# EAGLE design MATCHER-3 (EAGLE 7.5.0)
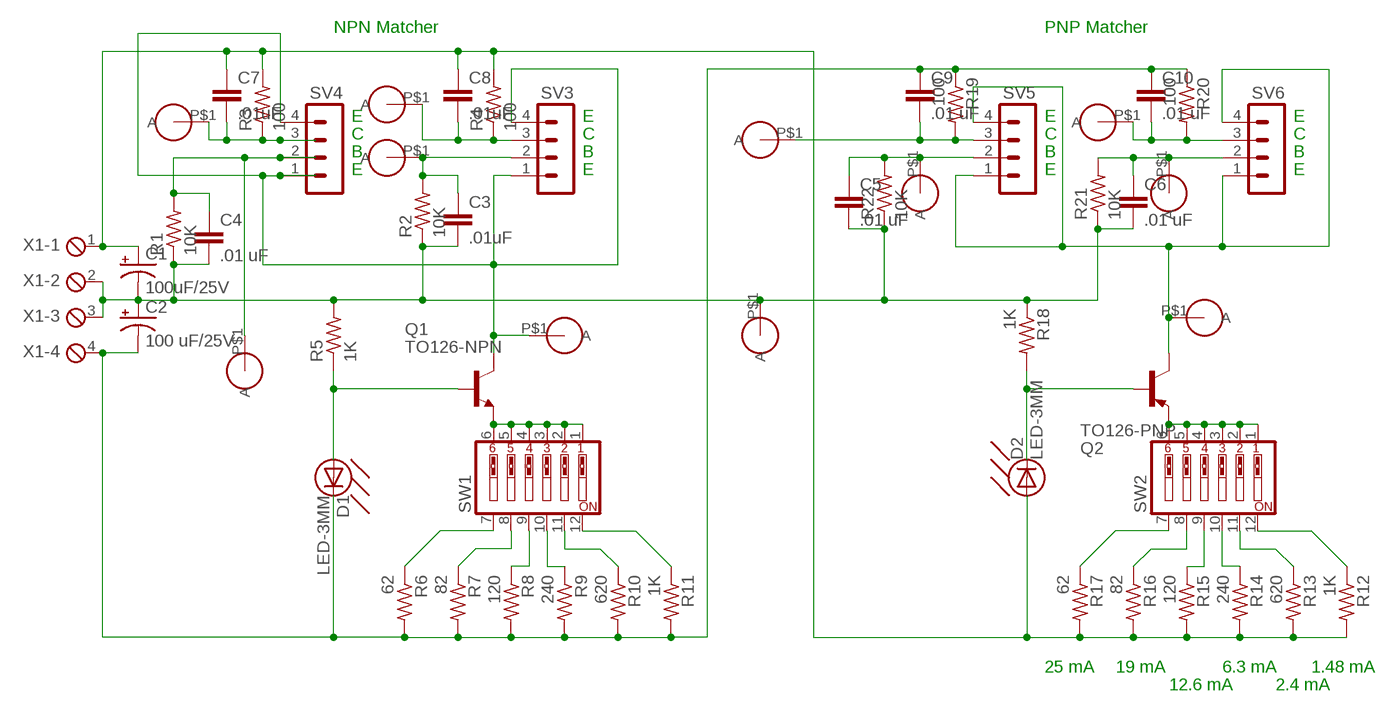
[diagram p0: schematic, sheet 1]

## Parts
C1  100uF/25V  CAP-POL-5/10  [CAP-POL-5/10]
C2  100 uF/25V  CAP-POL-5/10  [CAP-POL-5/10]
C3  .01uF  C5/2.5  [C5B2.5]
C4  .01 uF  C5/2.5  [C5B2.5]
C5  .01 uF  C5/2.5  [C5B2.5]
C6  .01 uF  C5/2.5  [C5B2.5]
C7  .01uF  C5/2.5  [C5B2.5]
C8  .01uF  C5/2.5  [C5B2.5]
C9  .01 uF  C5/2.5  [C5B2.5]
C10  .01 uF  C5/2.5  [C5B2.5]
D1  LED-3MM  [LED3MM]
D2  LED-3MM  [LED3MM]
GND  TESTPOINT  [TEST]
Q1  TO126-NPN  [TO126]
Q2  TO126-PNP  [TO126]
R1  10K  RESISTOR-1/4W  [FILM-RESISTOR]
R2  10K  RESISTOR-1/4W  [FILM-RESISTOR]
R3  100  RESISTOR-1/4W  [FILM-RESISTOR]
R4  100  RESISTOR-1/4W  [FILM-RESISTOR]
R5  1K  RESISTOR-1/4W  [FILM-RESISTOR]
R6  62  RESISTOR-1/4W  [FILM-RESISTOR]
R7  82  RESISTOR-1/4W  [FILM-RESISTOR]
R8  120  RESISTOR-1/4W  [FILM-RESISTOR]
R9  240  RESISTOR-1/4W  [FILM-RESISTOR]
R10  620  RESISTOR-1/4W  [FILM-RESISTOR]
R11  1K  RESISTOR-1/4W  [FILM-RESISTOR]
R12  1K  RESISTOR-1/4W  [FILM-RESISTOR]
R13  620  RESISTOR-1/4W  [FILM-RESISTOR]
R14  240  RESISTOR-1/4W  [FILM-RESISTOR]
R15  120  RESISTOR-1/4W  [FILM-RESISTOR]
R16  82  RESISTOR-1/4W  [FILM-RESISTOR]
R17  62  RESISTOR-1/4W  [FILM-RESISTOR]
R18  1K  RESISTOR-1/4W  [FILM-RESISTOR]
R19  100  RESISTOR-1/4W  [FILM-RESISTOR]
R20  100  RESISTOR-1/4W  [FILM-RESISTOR]
R21  10K  RESISTOR-1/4W  [FILM-RESISTOR]
R22  10K  RESISTOR-1/4W  [FILM-RESISTOR]
SV3  MA04-1  [MA04-1]
SV4  MA04-1  [MA04-1]
SV5  MA04-1  [MA04-1]
SV6  MA04-1  [MA04-1]
SW1  SW_DIP-6  [EDG-06]
SW2  SW_DIP-6  [EDG-06]
VB-A-N  TESTPOINT  [TEST]
VB-A-P  TESTPOINT  [TEST]
VB-B-N  TESTPOINT  [TEST]
VB-B-P  TESTPOINT  [TEST]
VC-A-N  TESTPOINT  [TEST]
VC-A-P  TESTPOINT  [TEST]
VC-B-N  TESTPOINT  [TEST]
VC-B-P  TESTPOINT  [TEST]
VE-N  TESTPOINT  [TEST]
VE-P  TESTPOINT  [TEST]
X1  MPT4  [4POL254]

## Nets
GND: C1.P$2(-) C2.P$1(+) C3.2 C4.2 C5.2 C6.2 GND.P$1(A) R1.P$1 R2.P$1 R5.P$2 R18.P$1 R21.P$1 R22.P$1 X1.2 X1.3
N$1: Q1.1(E) SW1.1 SW1.2 SW1.3 SW1.4 SW1.5 SW1.6
N$2: R6.P$1 SW1.7
N$3: R11.P$1 SW1.12
N$4: R8.P$1 SW1.9
N$5: R7.P$1 SW1.8
N$6: R9.P$1 SW1.10
N$7: R10.P$1 SW1.11
N$8: C5.1 R22.P$2 SV5.2 VB-A-P.P$1(A)
N$9: R15.P$1 SW2.9
N$10: D1.P$1-A(A) Q1.3(B) R5.P$1
N$11: Q1.2(C) SV3.1 SV3.4 SV4.1 SV4.4 VE-N.P$1(A)
N$12: C9.2 R19.P$2 SV5.3 VC-A-P.P$1(A)
N$13: C3.1 R2.P$2 SV3.2 VB-B-N.P$1(A)
N$14: C7.2 R3.P$1 SV4.3 VC-A-N.P$1(A)
N$15: C4.1 R1.P$2 SV4.2 VB-A-N.P$1(A)
N$16: C8.2 R4.P$1 SV3.3 VC-B-N.P$1(A)
N$17: C1.P$1(+) C7.1 C8.1 D2.P$1-A(A) R3.P$2 R4.P$2 R12.P$2 R13.P$2 R14.P$2 R15.P$2 R16.P$2 R17.P$2 X1.1
N$18: R14.P$1 SW2.10
N$19: R13.P$1 SW2.11
N$20: R12.P$1 SW2.12
N$21: R17.P$1 SW2.7
N$22: R16.P$1 SW2.8
N$23: Q2.1(E) SW2.1 SW2.2 SW2.3 SW2.4 SW2.5 SW2.6
N$26: C2.P$2(-) C9.1 C10.1 D1.P$2-C(C) R6.P$2 R7.P$2 R8.P$2 R9.P$2 R10.P$2 R11.P$2 R19.P$1 R20.P$1 X1.4
N$27: C6.1 R21.P$2 SV6.2 VB-B-P.P$1(A)
N$28: C10.2 R20.P$2 SV6.3 VC-B-P.P$1(A)
N$29: Q2.2(C) SV5.1 SV5.4 SV6.1 SV6.4 VE-P.P$1(A)
N$32: D2.P$2-C(C) Q2.3(B) R18.P$2

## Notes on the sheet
- NPN Matcher | PNP Matcher
- E | E | E | E
- C | C | C | C
- B | B | B | B
- E | E | E | E
- 25 mA | 19 mA | 6.3 mA | 1.48 mA
- 12.6 mA | 2.4 mA

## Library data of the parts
C1 C2 = ADC Project:CAP-POL-5/10
C3-C10 = capacitor-wima:C: CAPACITOR
D1 D2 = Adcom Project:LED-3MM
GND VB-A-N VB-A-P VB-B-N VB-B-P VC-A-N VC-A-P VC-B-N VC-B-P VE-N VE-P = Adcom Project:TESTPOINT
Q1 = Adcom Project:TO126-NPN
Q2 = Adcom Project:TO126-PNP
R1-R22 = ADC Project:RESISTOR-1/4W: 1/4 Watt Resistor
SV3-SV6 = con-lstb:MA04-1: PIN HEADER; OC_FARNELL: unknown; OC_NEWARK: unknown
SW1 SW2 = special:SW_DIP-6: DIP SWITCH
X1 = con-phoenix-254:MPT4: PHOENIX CONNECTOR; OC_FARNELL: unknown; OC_NEWARK: unknown

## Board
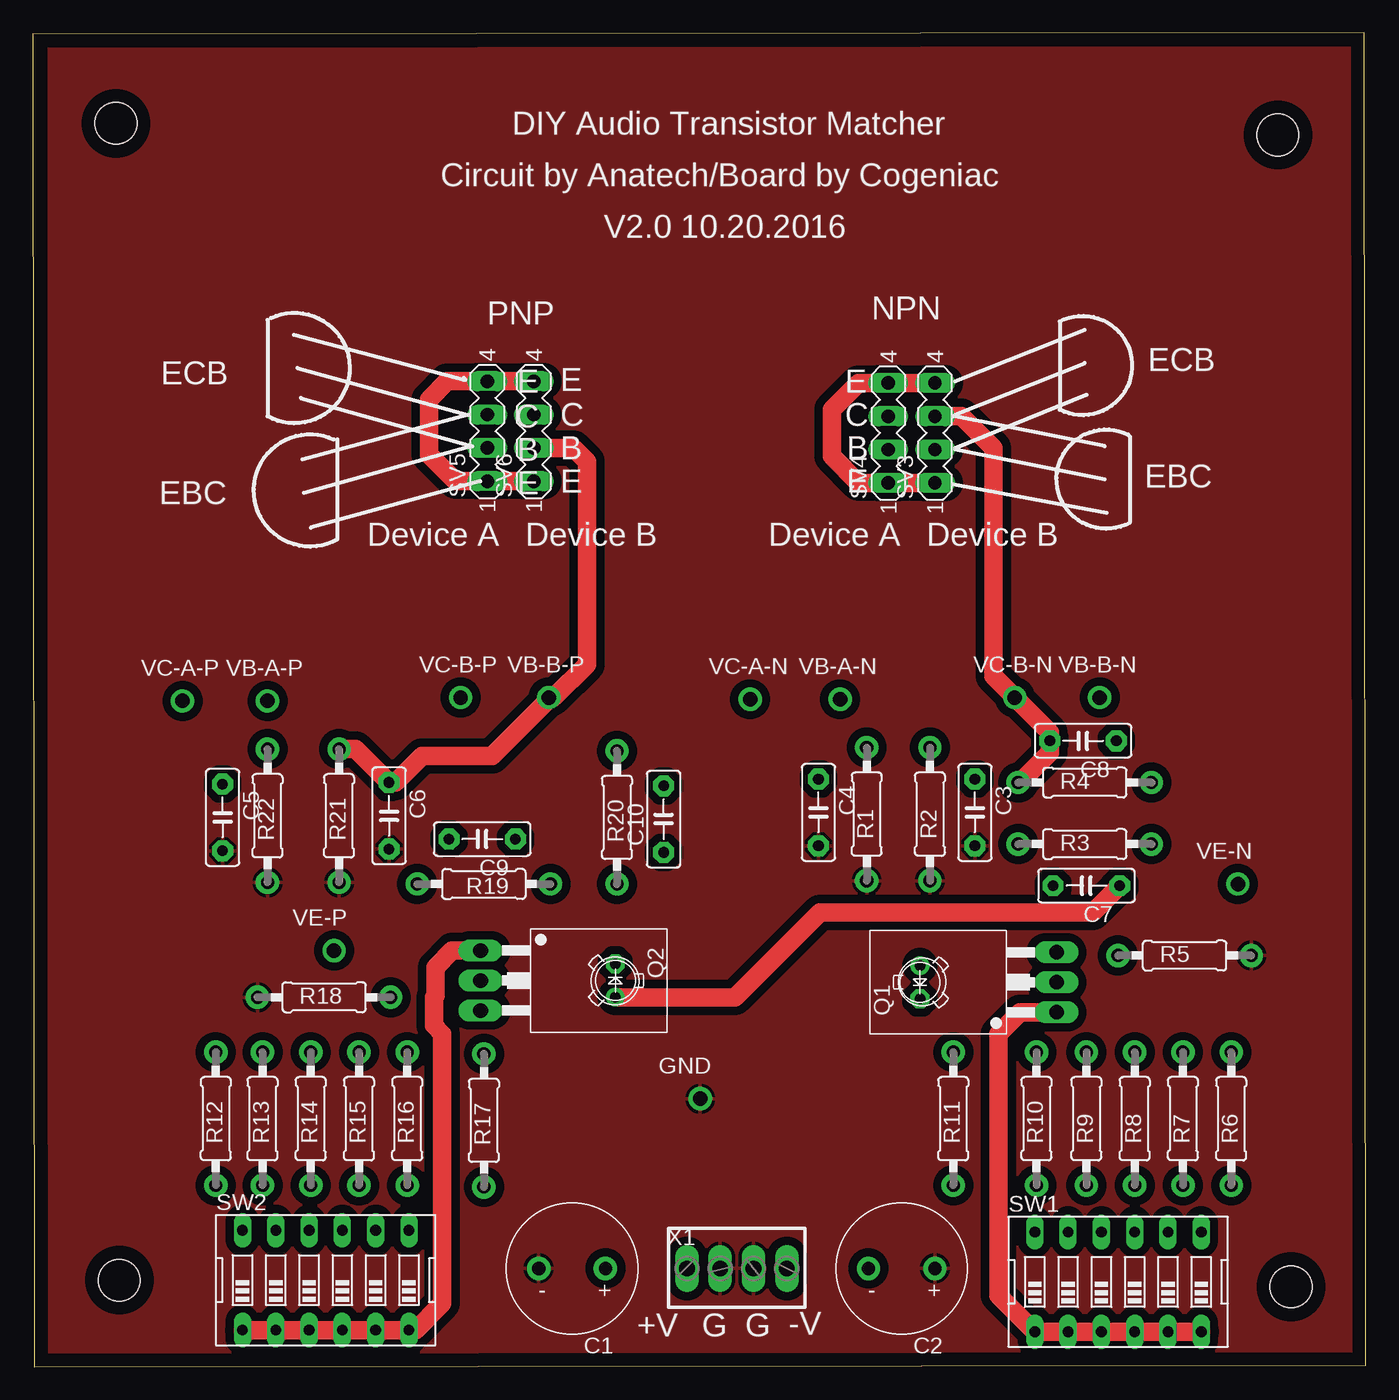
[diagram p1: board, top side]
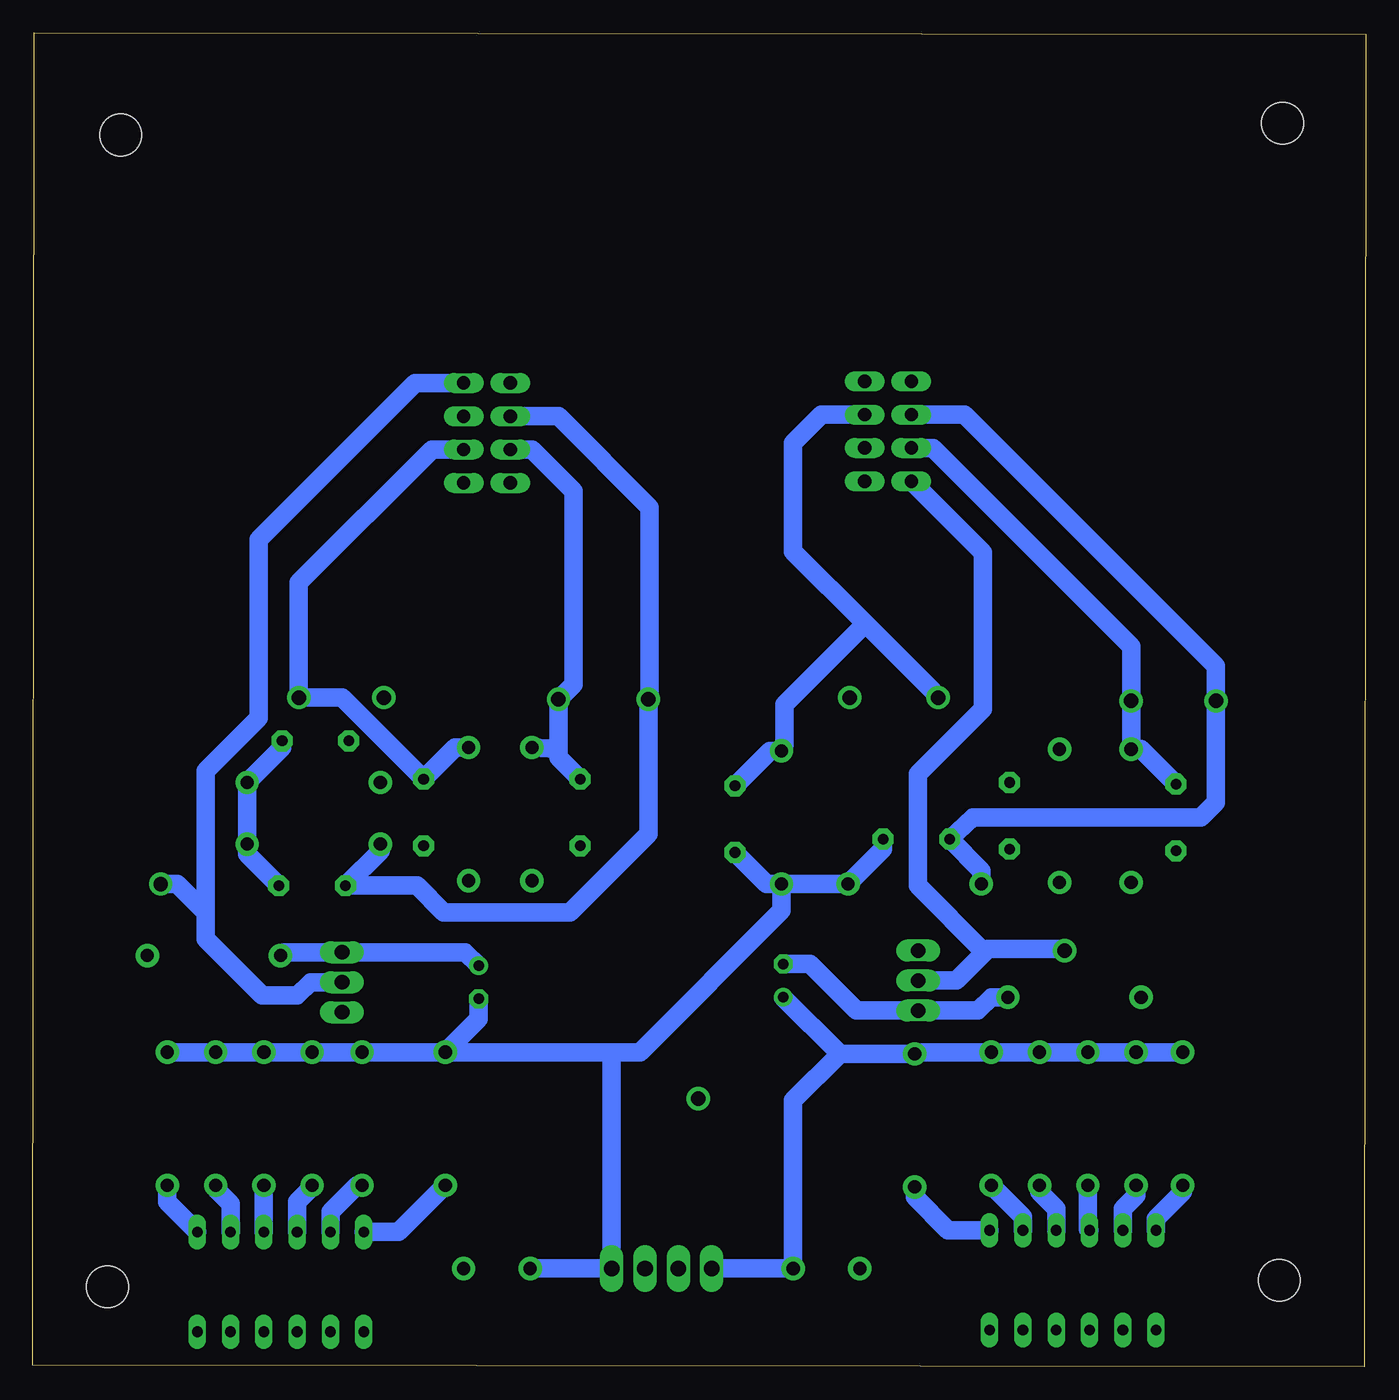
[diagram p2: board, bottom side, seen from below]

Size 101.71 x 101.78 mm. Coordinates in mm from the lower left corner, seen from the top.
Outline: 0.13,0 101.71,0.13 101.58,101.78 0,101.65 0.13,0
Copper layers (1*16): Top 0.035mm / dielectric 1.5mm / Bottom 0.035mm
Design rules "default *": minimum track width 56mil, minimum drill 24mil, track to track 25mil, track to pad 15mil, pad to pad 15mil, via to via 8mil, smd to smd 8mil, copper to edge 40mil, drill to drill 8mil, minimum pad ring 10mil, minimum via ring 8mil, stop-mask expansion 4mil, vias tented up to drill 0mil, thermal gap 10mil
Holes 3.2 mm at 6.6,6.6 6.35,94.87 95,93.98 96.01,6.1

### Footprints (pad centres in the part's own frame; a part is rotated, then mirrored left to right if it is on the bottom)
CAP-POL-5/10 = drill 1 pad 1.778: P$1 -2.54,0; P$2 2.54,0
C5B2.5 = drill 0.813 pad 1.6 octagon: 1 -2.54,0; 2 2.54,0
LED3MM = drill 0.8 pad 1.422: P$1-A 0,-1.27 | drill 0.8 pad 1.422 octagon: P$2-C 0,1.27
TEST = drill 1.1 pad 1.778: P$1 0,0
TO126 = drill 1.118 long: 1 -2.286,-6.35; 2 0,-6.35; 3 2.286,-6.35
FILM-RESISTOR = drill 1 pad 1.778: P$1 -5.08,0; P$2 5.08,0
MA04-1 = drill 1.016 long: 1 -3.81,0; 2 -1.27,0; 3 1.27,0; 4 3.81,0
EDG-06 = drill 0.813 long: 1 -6.35,-3.81; 2 -3.81,-3.81; 3 -1.27,-3.81; 4 1.27,-3.81; 5 3.81,-3.81; 6 6.35,-3.81; 7 6.35,3.81; 8 3.81,3.81; 9 1.27,3.81; 10 -1.27,3.81; 11 -3.81,3.81; 12 -6.35,3.81
4POL254 = drill 1.2 long: 1 -3.81,0; 2 -1.27,0; 3 1.27,0; 4 3.81,0

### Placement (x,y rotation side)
C1  41.15,7.49 180 top
C2  66.29,7.49 180 top
C3  71.88,42.29 270 top
C4  59.94,42.29 270 top
C5  14.48,41.91 270 top
C6  27.18,42.04 270 top
C7  80.39,36.7 180 top
C8  80.14,47.75 180 top
C9  34.29,40.26 180 top
C10  48.13,41.78 90 top
D1  67.69,29.34 180 top
D2  44.45,29.46 0 top
GND  50.93,20.45 0 top
Q1  71.75,29.34 90 top
Q2  40.51,29.46 270 top
R1  63.63,42.16 90 top
R2  68.45,42.16 90 top
R3  80.26,39.88 0 top
R4  80.26,44.58 0 top
R5  87.88,31.37 0 top
R6  91.44,18.92 90 top
R7  87.76,18.92 90 top
R8  84.07,18.92 90 top
R9  80.39,18.92 90 top
R10  76.58,18.92 90 top
R11  70.23,18.92 90 top
R12  13.97,18.92 90 top
R13  17.53,18.92 90 top
R14  21.21,18.92 90 top
R15  24.89,18.92 90 top
R16  28.57,18.92 90 top
R17  34.42,18.8 90 top
R18  22.22,28.19 0 top
R19  34.42,36.83 180 top
R20  44.58,41.91 90 top
R21  23.37,42.04 90 top
R22  17.91,42.04 90 top
SV3  68.83,71.25 90 top
SV4  65.28,71.25 90 top
SV5  34.67,71.37 90 top
SV6  38.23,71.37 90 top
SW1  82.8,6.48 0 top
SW2  22.35,6.6 0 top
VB-A-N  61.6,50.93 0 top
VB-A-P  17.91,50.8 0 top
VB-B-N  81.41,51.05 0 top
VB-B-P  39.37,51.05 0 top
VC-A-N  54.74,50.93 0 top
VC-A-P  11.43,50.8 0 top
VC-B-N  74.93,51.05 0 top
VC-B-P  32.64,51.05 0 top
VE-N  91.95,36.83 0 top
VE-P  22.99,31.75 0 top
X1  53.72,7.49 0 top

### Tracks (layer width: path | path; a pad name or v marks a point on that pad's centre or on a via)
GND
  pour Top: 1.27,100.71 100.71,100.71 100.71,0.76 1.27,0.76
N$1
  Top 1.422: SW1.6 SW1.5 SW1.4 SW1.3 SW1.2 SW1.1 73.66,5.46 73.66,25.4 75.31,27.05 Q1.1
N$2
  Bottom 1.422: R6.P$1 91.44,12.57 SW1.7
N$3
  Bottom 1.422: SW1.12 73.79,10.29 R11.P$1
N$4
  Bottom 1.422: R8.P$1 SW1.9
N$5
  Bottom 1.422: R7.P$1 87.76,13.59 86.61,12.45 SW1.8
N$6
  Bottom 1.422: R9.P$1 80.39,13.72 81.53,12.57 SW1.10
N$7
  Bottom 1.422: R10.P$1 76.96,13.84 78.99,11.81 SW1.11
N$8
  Bottom 1.422: SV5.2 34.07,70.08 33.05,70.08 17.91,54.94 VB-A-P.P$1 R22.P$2 17.14,47.12 C5.1
N$9
  Bottom 1.422: R15.P$1 24.89,13.34 23.62,12.07 SW2.9
N$10
  Bottom 1.422: D1.P$1-A 68.71,31.62 Q1.3 82.55,31.62 R5.P$1
N$11
  Top 1.422: SV3.4 SV4.4 62.99,75.06 60.96,73.02 60.96,69.47 62.99,67.44 SV4.1 SV3.1
  Bottom 1.422: SV3.4 72.52,75.06 84.45,63.12 84.45,60.85 84.48,60.82 84.48,49.51 88.52,45.47 88.52,34.67 | 88.52,34.67 88.52,32.64 84.2,28.32 81.53,28.32 80.52,29.34 Q1.2 | VE-N.P$1 90.68,36.83 88.52,34.67
N$12
  Bottom 1.422: SV5.3 30.61,72.64 11.44,53.48 11.44,51.56 VC-A-P.P$1 11.44,50.53 11.44,43.04 12.57,41.91 29.97,41.91 C9.2 29.34,37.85 R19.P$2
N$13
  Bottom 1.422: SV3.2 71.25,69.98 81.41,59.82 VB-B-N.P$1 78.1,51.05 C3.1 69.47,47.24 R2.P$2
N$14
  Bottom 1.422: SV4.3 61.6,72.52 54.65,65.57 54.65,51.56 VC-A-N.P$1 54.74,40.64 60.71,34.67 70.36,34.67 72.39,36.7 C7.2 75.18,39.37 R3.P$1
N$15
  Bottom 1.422: SV4.2 63.63,69.98 60.45,66.8 60.45,52.07 VB-A-N.P$1 61.6,46.99 | 61.6,46.99 61.6,46.48 C4.1 | R1.P$2 61.72,47.12 61.6,46.99
N$16
  Top 1.422: R4.P$1 75.31,44.58 77.6,46.86 C8.2 77.6,48.39 VC-B-N.P$1 73.28,52.71 73.28,70.1 70.87,72.52 SV3.3
N$17
  Top 1.422: D2.P$1-A 53.59,28.19 60.07,34.67 80.9,34.67 C7.1
  Bottom 1.422: R12.P$2 R13.P$2 R14.P$2 R15.P$2 R16.P$2 34.29,24 R17.P$2 40.13,23.88 | 40.13,23.88 D2.P$1-A | 40.13,23.88 43.69,20.32 C1.P$1 X1.1 | C8.1 82.68,47.24 R4.P$2 R3.P$2 85.34,39.12 C7.1
N$18
  Bottom 1.422: R14.P$1 21.21,10.54 SW2.10
N$19
  Bottom 1.422: R13.P$1 17.53,13.08 18.54,12.07 SW2.11
N$20
  Bottom 1.422: R12.P$1 13.97,13.34 16,11.3 SW2.12
N$21
  Bottom 1.422: R17.P$1 34.42,12.95 31.88,10.41 SW2.7
N$22
  Bottom 1.422: R16.P$1 26.16,11.43 SW2.8
N$23
  Top 1.422: SW2.1 SW2.2 SW2.3 SW2.4 SW2.5 SW2.6 29.21,2.79 31.24,4.83 31.24,25.4 30.61,26.04 30.61,28.19 30.73,28.32 30.73,30.48 32,31.75 Q2.1
N$26
  Bottom 1.422: R20.P$1 44.58,34.8 55.37,24 57.66,24 | 57.66,24 R11.P$2 | R11.P$2 R10.P$2 R9.P$2 R8.P$2 R7.P$2 R6.P$2 | C9.1 36.83,39.5 R19.P$1 R20.P$1 | R20.P$1 45.72,36.83 C10.1 | C2.P$2 X1.4 57.53,23.88 57.66,24 | D1.P$2-C 67.69,26.54 R11.P$2
N$27
  Top 1.422: SV6.2 39.22,70.08 41.28,70.08 42.3,69.05 42.3,54.65 42.29,54.64 42.29,53.59 39.75,51.05 VB-B-P.P$1 39.37,50.93 35.05,46.61 29.72,46.61 27.69,44.58 C6.1 24.64,47.12 R21.P$2
N$28
  Bottom 1.422: 38.19,56.71 33.05,51.56 VC-B-P.P$1 | 38.19,56.71 43.69,62.21 43.69,70.48 41.53,72.64 SV6.3 | 38.19,56.71 44.36,50.53 44.36,47.45 R20.P$2 45.47,46.99 C10.2
N$29
  Top 1.422: SV6.1 SV5.1 32.26,67.56 30.23,69.6 30.23,73.79 31.62,75.18 SV5.4 SV6.4
  Bottom 1.422: SV5.1 29.21,62.1 29.21,50.16 34.16,45.21 34.16,36.7 29.08,31.62 | Q2.2 31.24,29.46 29.08,31.62 | 29.08,31.62 28.83,31.88 23.11,31.88 VE-P.P$1
N$32
  Bottom 1.422: R18.P$2 28.57,28.19 29.59,27.18 Q2.3 38.86,27.18 42.42,30.73 D2.P$2-C

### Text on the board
tPlace: V2.0 10.20.2016 | ECB | ECB | EBC | EBC | Device A | Device B | Device A | Device B | +V | G | G | -V
tNames: DIY Audio Transistor Matcher | Circuit by Anatech/Board by Cogeniac | NPN | PNP | E | E | E | C | C | C | B | B | B | E | E | E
